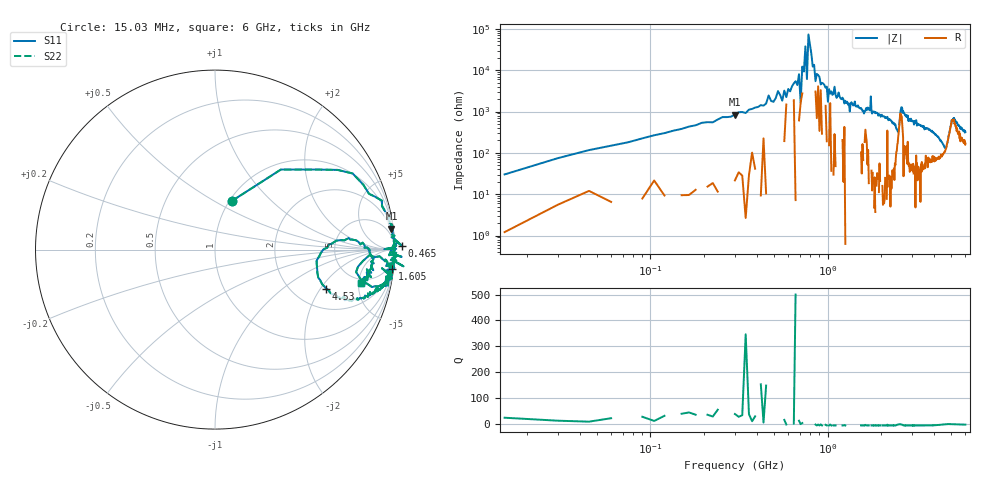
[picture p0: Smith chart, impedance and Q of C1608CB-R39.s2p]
!	Network	Analyzer	HP8753E.07.74:	Oct	30	2002	Serial	No.	JP38451487
!	Hewlett-Packard
!	27	Aug	2009	14:32:52
!	Frequency	S11	S21	S12	S22
#	HZ	S	RI	R	50
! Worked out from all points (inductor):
!   400 points, 15.03 MHz to 6 GHz, reference 50 ohm
!   read as one part in series: L = 391 nH near 45.03 MHz
!   highest Q = 38.4 at 300 MHz (marker M1), where L = 448 nH
!   self-resonance near 570 MHz
!   S11 on the Smith chart (normalised r, x): 15.03 MHz: 1.02, +0.60; 465 MHz: -39, +21; 1.605 GHz: 1, -18; 4.53 GHz: 2.95, -2.26; 6 GHz: 4.38, -5.43
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1.502992e7  0.0925 0.27  0.908 -0.27  0.908 -0.27  0.0925 0.27
9.002955e7  0.826 0.362  0.174 -0.362  0.174 -0.362  0.826 0.362
3.000285e8  0.983 0.116  0.0167 -0.116  0.0167 -0.116  0.983 0.116
4.650277e8  1.04 0.0227  -0.0359 -0.0227  -0.0359 -0.0227  1.04 0.0227
6.900266e8  0.999 0.0124  0.0011 -0.0124  0.0011 -0.0124  0.999 0.0124
7.050265e8  0.943 0.00259  0.0575 -0.00259  0.0575 -0.00259  0.943 0.00259
7.200264e8  0.998 0.00793  0.00189 -0.00793  0.00189 -0.00793  0.998 0.00793
7.350263e8  1.01 0.00372  -0.0102 -0.00372  -0.0102 -0.00372  1.01 0.00372
7.500262e8  1 0.00262  -0.00036 -0.00262  -0.00036 -0.00262  1 0.00262
7.650262e8  0.994 0.0152  0.00583 -0.0152  0.00583 -0.0152  0.994 0.0152
7.800261e8  1 -0.00122  -0.00061 0.00122  -0.00061 0.00122  1 -0.00122
8.550257e8  0.989 -0.0149  0.0105 0.0149  0.0105 0.0149  0.989 -0.0149
1.020025e9  0.998 -0.0286  0.00208 0.0286  0.00208 0.0286  0.998 -0.0286
1.605022e9  0.988 -0.11  0.0122 0.11  0.0122 0.11  0.988 -0.11
1.755021e9  1 -0.043  -0.0014 0.043  -0.0014 0.043  1 -0.043
1.785021e9  0.986 -0.11  0.0138 0.11  0.0138 0.11  0.986 -0.11
2.01002e9  0.984 -0.122  0.016 0.122  0.016 0.122  0.984 -0.122
3.015015e9  0.978 -0.166  0.022 0.166  0.022 0.166  0.978 -0.166
4.00501e9  0.851 -0.264  0.149 0.264  0.149 0.264  0.851 -0.264
4.530007e9  0.619 -0.218  0.381 0.218  0.381 0.218  0.619 -0.218
5.010005e9  0.848 0.0123  0.152 -0.0123  0.152 -0.0123  0.848 0.0123
6e9  0.816 -0.186  0.184 0.186  0.184 0.186  0.816 -0.186
